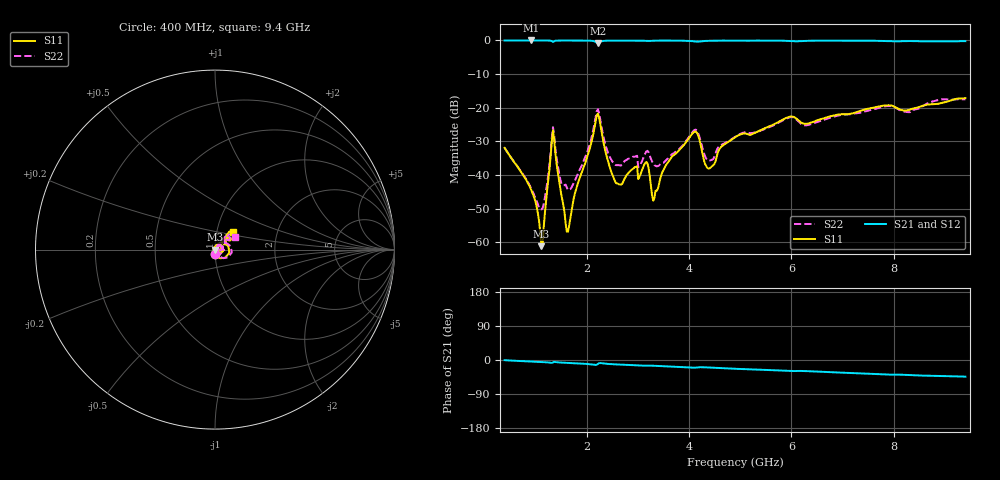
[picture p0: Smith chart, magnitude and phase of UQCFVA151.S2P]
!  Part Number  UQCFVA151  Mounting Orientation: Horizontal
!  Description: Ultra Low ESR Microwave capacitors
!  Application: Coupling, Bypass, Tuning, DC Block
!  Filters, Matching
# GHZ S DB R 50
! Freq  |S11|  S11 Ph  |S21|  S21 Ph  |S12|  S12 Ph  |S22|  S22 Ph
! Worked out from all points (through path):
!   401 points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, 400 MHz to 9.4 GHz, reference 50 ohm
!   highest |S21| = 0.00 dB at 918 MHz (marker M1); lowest = -0.8 dB at 2.223 GHz (marker M2)
!   group delay of S21, straight-line fit = 13.4 ps
!   lowest |S11| = -61.1 dB at 1.12 GHz (marker M3), VSWR 1.00, Z = 49.9 - j0.0232 ohm
!   |S11| at or under -10 dB: start of sweep to end of sweep
!   |S22| runs from -50.2 to -17.4 dB; largest |S21 - S12| = 0.0029
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0.4  -31.92 -89.3  -0.01 -0.5  0.00 -0.5  -31.90 -88.1
0.918  -44.36 -98.9  0.00 -4.0  0.00 -4.0  -43.96 -72.6
1.12  -61.14 -164.6  -0.01 -5.3  -0.01 -5.3  -50.23 -7.0
1.165  -55.30 110.7  -0.01 -5.6  -0.01 -5.6  -48.49 23.4
1.3  -34.27 58.5  -0.09 -7.2  -0.08 -7.2  -32.99 50.5
1.345  -26.72 -10.1  -0.44 -6.4  -0.43 -6.3  -25.77 -3.9
1.503  -45.45 -113.4  -0.02 -6.8  -0.02 -6.8  -42.24 -48.5
1.638  -56.84 -172.2  -0.02 -7.7  -0.02 -7.7  -44.47 -11.0
1.908  -39.17 95.7  -0.03 -9.6  -0.02 -9.5  -37.13 44.6
2.223  -21.73 -12.8  -0.81 -10.3  -0.80 -10.2  -20.45 -9.9
2.425  -36.17 -107.6  -0.06 -10.4  -0.06 -10.4  -33.70 -52.8
2.583  -42.46 -137.4  -0.06 -11.7  -0.05 -11.7  -37.07 -24.7
3.145  -36.40 37.4  -0.12 -15.1  -0.12 -15.1  -33.63 24.4
3.303  -47.62 26.3  -0.07 -15.1  -0.07 -15.1  -36.60 3.7
3.415  -42.77 73.5  -0.04 -15.9  -0.04 -15.9  -37.20 23.5
4.09  -27.32 32.0  -0.26 -20.2  -0.26 -20.2  -26.86 30.8
4.383  -38.07 24.2  -0.11 -19.9  -0.10 -19.8  -35.73 23.2
4.9  -28.81 54.9  -0.04 -23.1  -0.04 -23.1  -28.67 56.5
5.98  -22.61 37.5  -0.18 -29.2  -0.18 -29.1  -22.80 48.0
6.408  -24.30 40.3  -0.08 -30.0  -0.08 -30.0  -24.79 51.6
7.915  -19.27 35.1  -0.20 -38.5  -0.21 -38.5  -19.51 41.0
9.4  -17.16 43.4  -0.21 -43.9  -0.21 -43.9  -17.51 31.5
